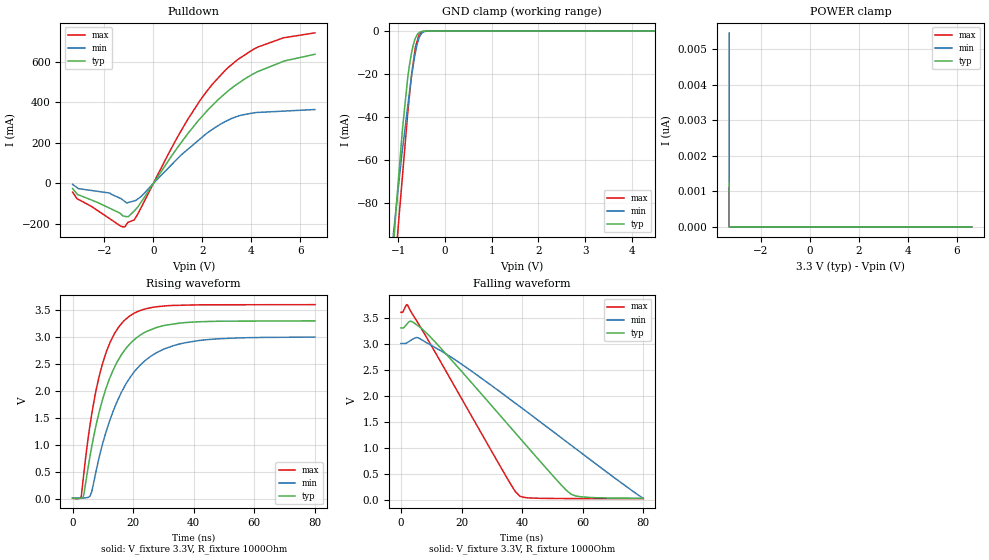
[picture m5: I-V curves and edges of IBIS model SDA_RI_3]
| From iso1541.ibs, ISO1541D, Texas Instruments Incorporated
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|   SDA Right 3.3V I/O Model
[Model]   SDA_RI_3
Model_type   I/O_open_drain
Polarity   Non-Inverting
Enable   Active-Low
Vinl = 0.9
Vinh = 2.52
Vmeas = 1.65
Vref = 1.65
Cref = 15pF
Rref = 1000
|   typ   min   max
|   (nom PVT)   (fast PVT)   (slow PVT)
C_comp   1.957p   1.640p   2.653p
|C_comp (ON state)   1.957p   1.640p   2.653p
|C_comp (OFF state)   4.105p   3.069p   5.182p
|PVT   Nom   Slow   Fast
[Voltage Range]   3.3   3   3.6
[Temperature Range]   27   136   -40
[Pullup Reference]   3.3   3   3.6
[Pulldown Reference]   -0   -0   -0
[Power Clamp Reference]   3.3   3   3.6
[GND Clamp Reference]   -0   -0   -0
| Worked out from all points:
|   slope of the pulldown table from 0 to 0.495 V, typ, clamps not added: 5.5 ohm
|   GND clamp passes 1 mA (typ) near -0.56 V on its own axis
|   falling waveform, V_fixture 3.3V, R_fixture 1000Ohm: 20-80 % time 29.5ns typ, 41ns min, 21.1ns max; typ from 3.3 V to 0.023 V
|   rising waveform, V_fixture 3.3V, R_fixture 1000Ohm: 20-80 % time 10.4ns typ, 12.9ns min, 8.02ns max; typ from 0.018 V to 3.3 V
[Pulldown]
|   Voltage   I(typ)   I(min)   I(max)
-3.3V     -25.45mA   -4.956mA   -43.12mA
-3.115V   -52.44mA   -21.31mA   -76.35mA
-1.778V   -122.9mA   -47.71mA   -174.6mA
-1.163V   -162.6mA   -89.49mA   -214.4mA
-1.026V   -164.4mA   -94.36mA   -191.6mA
-629.9mV  -115.6mA   -76.18mA   -150.1mA
1.395V    243.6mA    166.8mA    313.9mA
2.16V     353.6mA    245.2mA    451.2mA
2.925V    442.8mA    304.5mA    556.7mA
4.271V    551.8mA    350.1mA    672.8mA
5.31V     602.1mA    356.5mA    718.1mA
6.6V      637.1mA    364.5mA    742.8mA
[GND Clamp]
|   Voltage   I(typ)   I(min)   I(max)
-3.3V     -759.2mA   -570.2mA   -927.9mA
-1.142V   -112.7mA   -103.6mA   -137.6mA
-1.078V   -93.5mA    -89.71mA   -115.2mA
-1.002V   -71.26mA   -74.08mA   -92.05mA
-909.3mV  -46.13mA   -55.48mA   -68.05mA
-794.9mV  -21.68mA   -35.16mA   -38.3mA
-755.4mV  -15.47mA   -28.13mA   -29.6mA
-709.8mV  -9.809mA   -20.52mA   -19.87mA
-629.9mV  -3.29mA    -9.977mA   -7.425mA
-524.4mV  -338uA     -1.998mA   -1.07mA
-327.3mV  -31.85uA   -19.07uA   -2.263uA
6.6V      0A         0A         0A
[POWER Clamp]
|   Voltage   I(typ)   I(min)   I(max)
-3.3V     1.227nA    5.456nA    1.121nA
-3.3V     0A         0A         0A
-3.3V     0A         0A         0A
6.6V      0A         0A         0A
[Ramp]
R_load = 1000
|   typ   min   max
dV/dt_r   1.96937/1.04301e-08   1.78574/1.29228e-08   2.15107/8.02123e-09
dV/dt_f   1.96592/2.94956e-08   1.78636/4.10048e-08   2.15033/2.1068e-08
[Falling Waveform]
V_fixture = 3.3V
V_fixture_min = 3V
V_fixture_max = 3.6V
R_fixture = 1000Ohm
C_fixture = 0F
|   Time   V(typ)   V(min)   V(max)
0s        3.3V       3V         3.6V
2.053ns   3.378V     3.016V     3.746V
3.441ns   3.425V     3.067V     3.6V
5.125ns   3.363V     3.115V     3.444V
6.988ns   3.279V     3.067V     3.264V
17.59ns   2.624V     2.699V     2.19V
34.49ns   1.5V       1.995V     467.7mV
39.29ns   1.179V     1.786V     61.85mV
56.27ns   98.33mV    1.04V      18.34mV
80ns      23.47mV    22.8mV     16.12mV
[Rising Waveform]
V_fixture = 3.3V
V_fixture_min = 3V
V_fixture_max = 3.6V
R_fixture = 1000Ohm
C_fixture = 0F
|   Time   V(typ)   V(min)   V(max)
0s        17.61mV    22.73mV    14.85mV
2.821ns   15.93mV    17.82mV    39.79mV
3.672ns   72.41mV    19.96mV    452mV
5.796ns   807mV      56.5mV     1.385V
10.04ns   1.871V     1.051V     2.537V
13.91ns   2.448V     1.698V     3.072V
18.49ns   2.846V     2.209V     3.376V
25.53ns   3.129V     2.633V     3.54V
36.73ns   3.266V     2.891V     3.59V
80ns      3.3V       2.999V     3.6V
